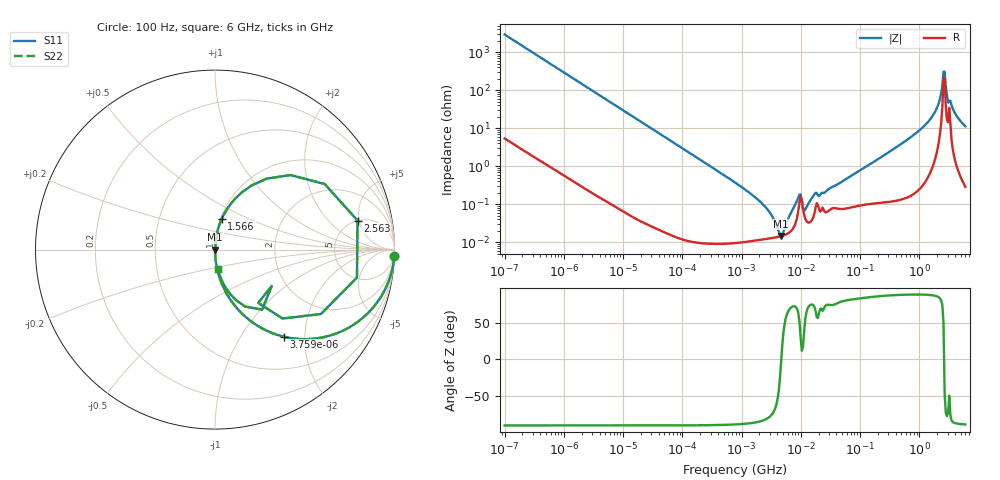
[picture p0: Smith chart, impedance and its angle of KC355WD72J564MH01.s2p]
!Murata Part Number: KC355WD72J564MH01
!These Parameters are Measured in Series Mode Connection
!Data Generated on Jun 19, 2026
!  o--ll--o
!Port1  Port2
!  o------o
!Operation Temp=25[degC], DC Bias Voltage=0[V]
!Freq. Start=100[Hz] Stop=6[GHz] 401[Steps]
# Hz S RI R 50
!Freq.(Hz) S11(Real) S11(Imag) S21(Real) S21(Imag) S12(Real) S12(Imag) S22(Real) S22(Imag)
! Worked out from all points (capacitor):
!   401 points, 100 Hz to 6 GHz, reference 50 ohm
!   read as one part in series: C = 540 nF near 109 Hz
!   lowest |Z| = 14.4 mohm at 4.644 MHz (marker M1)
!   series resonance near 4.681 MHz, so ESL is about 2.1 nH
!   S11 on the Smith chart (normalised r, x): 100 Hz: 1, -59; 3.759 kHz: 1.00, -1.57; 1.566 GHz: 1.01, +0.36; 2.563 GHz: 5.01, +4.72; 6 GHz: 1.01, -0.22
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100  0.9988 -0.0339  0.00121 0.0339  0.00121 0.0339  0.9988 -0.0339
717  0.9438 -0.2293  0.0562 0.2293  0.0562 0.2293  0.9438 -0.2293
2008  0.6835 -0.4641  0.3165 0.4641  0.3165 0.4641  0.6835 -0.4641
3759  0.3824 -0.485  0.6176 0.485  0.6176 0.485  0.3824 -0.485
9626  0.0869 -0.2806  0.9131 0.2806  0.9131 0.2806  0.0869 -0.2806
40335  0.00558 -0.0731  0.9944 0.0731  0.9944 0.0731  0.00558 -0.0731
774597  0.000108 -0.00372  0.9999 0.00372  0.9999 0.00372  0.000108 -0.00372
2481164  0.00012 -0.000859  0.9999 0.000859  0.9999 0.000859  0.00012 -0.000859
4643984  0.000143 -1.04e-05  0.9999 1.04e-05  0.9999 1.04e-05  0.000143 -1.04e-05
9090158  0.000688 0.00134  0.9993 -0.00134  0.9993 -0.00134  0.000688 0.00134
1.189169e7  0.000413 0.000586  0.9996 -0.000586  0.9996 -0.000586  0.000413 0.000586
1.555665e7  0.00039 0.00143  0.9996 -0.00143  0.9996 -0.00143  0.00039 0.00143
3.124326e8  0.00171 0.0237  0.9983 -0.0237  0.9983 -0.0237  0.00171 0.0237
8.749838e8  0.00738 0.0729  0.9926 -0.0729  0.9926 -0.0729  0.00738 0.0729
1.565993e9  0.0382 0.1724  0.9618 -0.1724  0.9618 -0.1724  0.0382 0.1724
1.95892e9  0.1114 0.2827  0.8886 -0.2827  0.8886 -0.2827  0.1114 0.2827
2.240541e9  0.2877 0.3953  0.7123 -0.3953  0.7123 -0.3953  0.2877 0.3953
2.562649e9  0.7943 0.1617  0.2057 -0.1617  0.2057 -0.1617  0.7943 0.1617
2.802721e9  0.59 -0.3589  0.41 0.3589  0.41 0.3589  0.59 -0.3589
3.065283e9  0.241 -0.2971  0.759 0.2971  0.759 0.2971  0.241 -0.2971
4.009986e9  0.0691 -0.2265  0.9309 0.2265  0.9309 0.2265  0.0691 -0.2265
6e9  0.0151 -0.11  0.9849 0.11  0.9849 0.11  0.0151 -0.11
